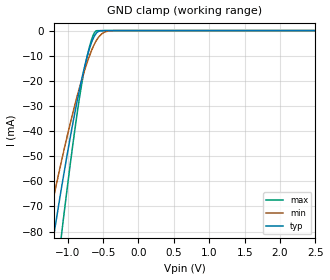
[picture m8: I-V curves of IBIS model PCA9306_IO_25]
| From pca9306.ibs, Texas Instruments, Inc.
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[Model]   PCA9306_IO_25
Model_type  Terminator
| variable   typ   min   max
C_comp   2.66pF   2.29pF   3.20pF
| C_tri-state   2.66pF   2.29pF   3.20pF
[Temperature Range]   40   100   -40
| Ambient temperature   25   85   -40
[Voltage range]   2.5   2.3   2.7
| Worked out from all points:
|   GND clamp passes 1 mA (typ) near -0.59 V on its own axis
[GND Clamp]
| PCA9306_IO_25
|   Voltage   I(typ)   I(min)   I(max)
-2.5V     -349.7mA   -272.4mA   -467.7mA
-1.315V   -103.2mA   -82.31mA   -137.3mA
-1.285V   -97.6mA    -78.12mA   -129.7mA
-1.2V     -82.18mA   -66.55mA   -108.4mA
-1.1V     -64.75mA   -53.5mA    -84.26mA
-1.075V   -60.52mA   -50.35mA   -78.37mA
-920mV    -35.84mA   -31.97mA   -43.85mA
-790mV    -17.89mA   -18.51mA   -19.31mA
-680mV    -6.109mA   -9.157mA   -5.225mA
-600mV    -1.21mA    -4.203mA   -179.9uA
-375mV    -1uA       -57.23uA   -10.78nA
2.5V      27.81pA    2.894nA    11.56pA
